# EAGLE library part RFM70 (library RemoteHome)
RFM70 2.4 Ghz Funkmodul Autor: Daniel Weber Website: http://projects.web4clans.com Email: daniel.weber@web4clans.com
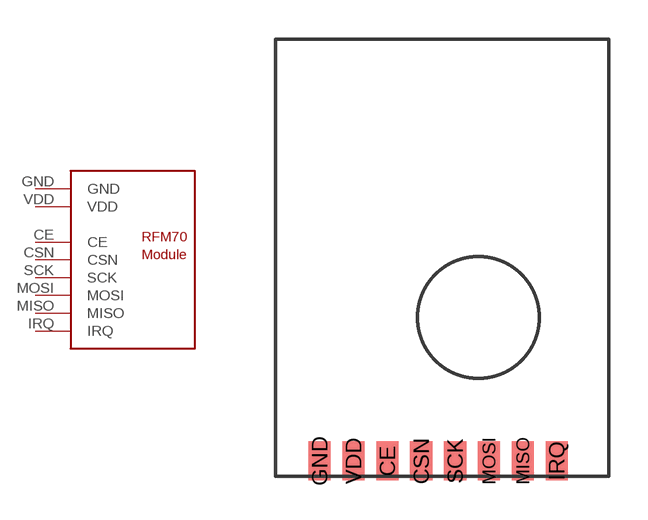
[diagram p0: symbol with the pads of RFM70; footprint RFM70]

Designator prefix -

## RFM70  [RFM70]
CE  CE
CSN  CSN
GND  GND  pwr
IRQ  IRQ
MISO  MISO
MOSI  MOSI
SCK  SCK
VDD  VDD  pwr

## Footprint RFM70 (pad centres in mm)
smd 0.85 x 1.5: CE 2.5,-14.3; CSN 3.8,-14.3; GND -0.1,-14.3; IRQ 9,-14.3; MISO 7.7,-14.3; MOSI 6.4,-14.3; SCK 5.1,-14.3; VDD 1.2,-14.3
